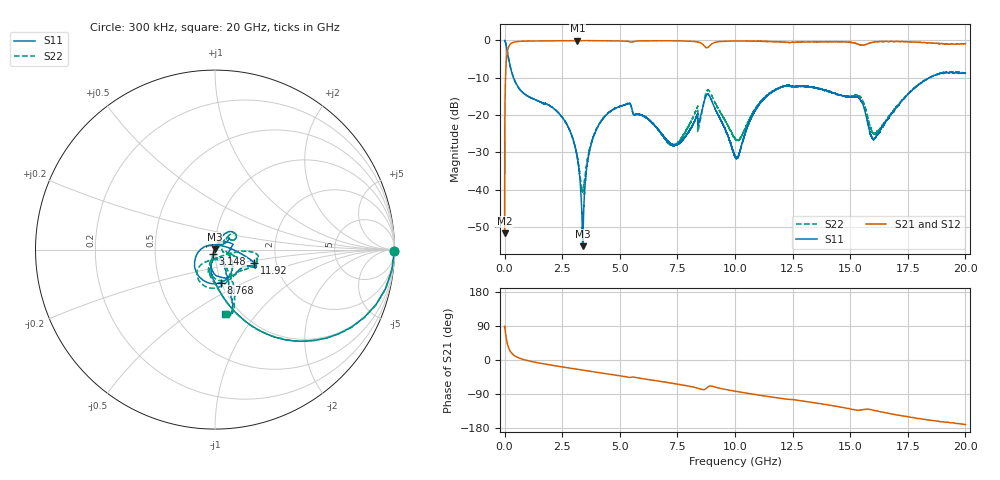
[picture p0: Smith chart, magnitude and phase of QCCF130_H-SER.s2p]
!{QCCF130}
!Johanson Technology Inc.
!www.johansontechnology.com
!Test Board Conditions:
!Substrate Type  RO4350B
!Substrate Thickness  10 mil
!Substrate Dk  3.66
!TL Type: GCPW
!TL Trace Width  21 mil
!TL Gap  20 mil
!Electrode orientation  Horizontal
!DUT TOPOLOGY	SERIES
!Mounting Pad LxW  16x21 mil
! Created Sat Jan  9 18:19:22 2021
# hz S ma R 50
! 2 Port Network Data from SP1.SP block
! freq  magS11  angS11  magS21  angS21  magS12  angS12  magS22  angS22
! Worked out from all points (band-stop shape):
!   20001 points, 300 kHz to 20 GHz, reference 50 ohm
!   highest |S21| = -0.03 dB at 3.156 GHz (marker M1); lowest = -51.7 dB at 300 kHz (marker M2)
!   |S21| within 3 dB of the highest: 119.7 MHz to end of sweep
!   lowest |S11| = -55.1 dB at 3.392 GHz (marker M3), VSWR 1.00, Z = 49.8 + j0.0729 ohm
!   |S11| at or under -10 dB: 389.7 MHz to 18.41 GHz (18.02 GHz wide, 192 % of centre); 18.41437 GHz to 18.42163 GHz (7.257 MHz wide, 0.0394 % of centre)
!   |S22| runs from -40.6 to 0.0 dB; largest |S21 - S12| = 0.013
!   S11 on the Smith chart (normalised r, x): 300 kHz: open; 3.148 GHz: 0.98, -0.05; 8.768 GHz: 0.99, -0.38; 11.92 GHz: 1.54, -0.24; 20 GHz: 0.85, -0.70
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300000  0.9986 -0.4  0.002599 86.1  0.002511 89.9  0.9994 -0.5
1.053e8  0.7466 -42.7  0.6596 47.2  0.661 47.1  0.7482 -42.5
2.323e8  0.4652 -64.8  0.8814 24.6  0.8811 24.6  0.4637 -64.9
2.5393e9  0.08985 -103.8  0.9927 -18.6  0.9919 -18.6  0.09002 -110.3
3.1483e9  0.02732 -112.0  0.9953 -24.3  0.9955 -24.4  0.02843 -101.7
3.1563e9  0.02651 -113.2  0.9969 -24.4  0.9956 -24.5  0.02748 -101.8
3.3343e9  0.006777 -126.7  0.9955 -26.1  0.9954 -26.1  0.01106 -64.2
3.3923e9  0.001751 155.3  0.9957 -26.7  0.9957 -26.7  0.009474 -27.3
3.7413e9  0.0389 68.9  0.9947 -30.0  0.9949 -30.0  0.04075 40.5
4.4013e9  0.0992 58.6  0.989 -36.2  0.9892 -36.1  0.1006 45.6
5.3863e9  0.143 39.8  0.9686 -45.6  0.9695 -45.5  0.1442 37.8
6.6673e9  0.06385 32.6  0.989 -55.5  0.9894 -55.5  0.06328 40.0
7.4223e9  0.03967 52.6  0.9871 -62.7  0.9876 -62.7  0.04001 -2.3
8.4873e9  0.0912 -25.1  0.9356 -76.4  0.9351 -76.4  0.08318 -23.1
8.7683e9  0.1869 -80.4  0.797 -74.3  0.7962 -74.2  0.206 -80.4
1.00003e10  0.02798 107.2  0.9839 -82.2  0.9821 -82.3  0.04838 -89.0
1.19173e10  0.2305 -18.7  0.9563 -100.6  0.9571 -100.6  0.2314 -6.0
1.33343e10  0.2364 -23.9  0.9539 -111.8  0.9553 -111.9  0.2358 -19.9
1.53653e10  0.1722 -67.7  0.8883 -132.5  0.8872 -132.3  0.1819 -73.3
1.60083e10  0.04759 -79.1  0.9474 -132.6  0.9477 -132.6  0.05638 -91.4
1.66673e10  0.08998 -59.2  0.9627 -140.6  0.9669 -140.9  0.09592 -59.4
2e10  0.3624 -80.9  0.9077 -170.4  0.9038 -170.4  0.3661 -80.2
